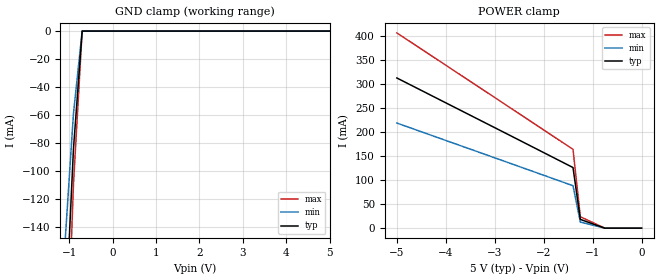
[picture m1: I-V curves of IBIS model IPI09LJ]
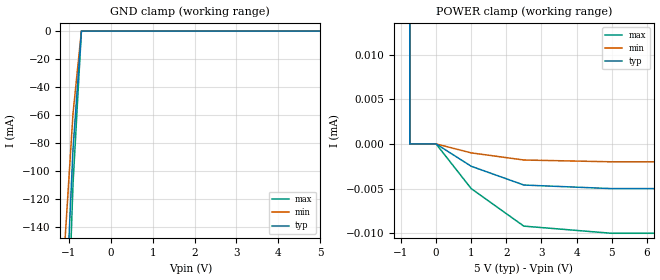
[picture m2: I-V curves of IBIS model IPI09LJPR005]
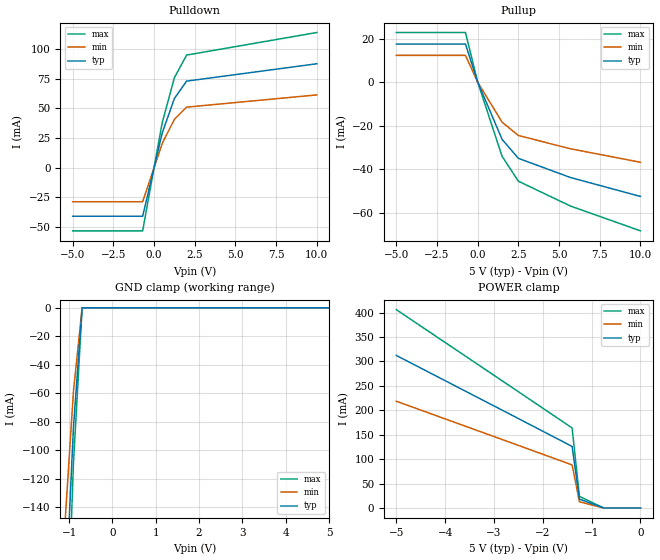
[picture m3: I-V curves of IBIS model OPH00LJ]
[IBIS Ver]   2.1
[File name]   act8997.ibs
[File Rev]   1.0   | from silicon model only
[Date]   97318
[Source]   Silicon-level model at Texas Instruments (ALEY)
[Notes]
   SCAN PATH LINKERS WITH 4-BIT IDENTIFICATION BUSES
   SCAN-CONTROLLED IEEE STD 1149.1 (JTAG) TAP CONCATENATORS
   Release 1.0) 97318 ALEY - initial release
   includes DCO open-drain (_OD) and DCO 3-state (_TS)
   includes all available commercial packages:
   DW=28SOIC (no-coupling model)
   NT=28PDIP (no-coupling model)
[Disclaimer]
   Property of Texas Instruments Incorporated.  Unauthorized
   reproduction and/or distribution is strictly prohibited.
   This product is protected under copyright law.
   Created 1997, (C) Copyright 1997, Texas Instruments Incorporated.
   All Rights Reserved
   UNLESS THERE IS A SIGNED, WRITTEN AGREEMENT TO THE
   CONTRARY, TEXAS INSTRUMENTS ("TI") IS PROVIDING THE IBIS
   MODELS "AS IS" AND WITHOUT ANY WARRANTY, EXPRESSED OR
   IMPLIED.  TI assumes no liability for:
   1) the accuracy of the IBIS models provided to your
   company;
   2) the proper functioning of these IBIS models in your
   design or for any resulting applications; or
   3) infringement of patents, copyrights or intellectual
   property rights resulting from your use of these IBIS
   models.
   TI provides IBIS Models as a service to our customers.
   You and your company shall not distribute, sell or give
   these models to anyone else without prior written
   permission from TI.
   TI reserves the right to make changes to our products or
   to discontinue any semiconductor product or service
   without notice, and advises our customers to obtain the
   latest version of relevant information to verify, before
   placing orders, that the information being relied on is
   current.
   Please be aware that your receipt and use of the IBIS
   information provided shall serve as acceptance of these
   terms and conditions.  If you do not accept these terms,
   you should return or destroy the IBIS models and any
   other accompanying information immediately.
[Component]   SN74ACT8997DW_OD
[Manufacturer]  Texas Instruments
[Package]
| 28-pin SOIC (suffix = DW)
| variable   typ   min   max
R_pkg   100m   NA   NA
L_pkg   7n   NA   NA
C_pkg   1p   NA   NA
[Pin]   signal_name   model_name   R_pin   L_pin   C_pin
1   DCO   OPHA1LJ   NA   8.15N   1.06P
2   MCO   OPH00LJ   NA   6.75N   0.98P
3   DTDO1   OPH03LJ   NA   5.49N   0.92P
4   DTDO2   OPH03LJ   NA   4.44N   0.64P
5   DTDO3   OPH03LJ   NA   3.74N   0.55P
6   DTDO4   OPH03LJ   NA   3.14N   0.46P
7   GND   GND   NA   2.85N   0.40P
8   DTMS1   OPHB3LJ   NA   2.85N   0.40P
9   DTMS2   OPHB3LJ   NA   3.14N   0.46P
10   DTMS3   OPHB3LJ   NA   3.74N   0.55P
11   DTMS4   OPHB3LJ   NA   4.44N   0.64P
12   DTCK   OPJE3LJ   NA   5.49N   0.92P
13   TDO   OPH03LJ   NA   6.75N   0.98P
14   TMS   IPI09LJPR005   NA   8.15N   1.06P
15   TCK   IPI09LJ   NA   8.15N   1.06P
16   TDI   IPI09LJPR005   NA   6.75N   0.98P
17   DTDI4   IPI09LJPR005   NA   5.49N   0.92P
18   DTDI3   IPI09LJPR005   NA   4.44N   0.64P
19   DTDI2   IPI09LJPR005   NA   3.74N   0.55P
20   DTDI1   IPI09LJPR005   NA   3.14N   0.46P
21   VCC   POWER   NA   2.85N   0.40P
22   ID4   IPI09LJ   NA   2.85N   0.40P
23   ID3   IPI09LJ   NA   3.14N   0.46P
24   ID2   IPI09LJ   NA   3.74N   0.55P
25   ID1   IPI09LJ   NA   4.44N   0.64P
26   TRSTN   IPI09LJPR005   NA   5.49N   0.92P
27   MCI   IPI09LJ   NA   6.75N   0.98P
28   DCI   IPI09LJ   NA   8.15N   1.06P
[Component]   SN74ACT8997DW_TS
[Manufacturer]  Texas Instruments
[Package]
| 28-pin SOIC (suffix = DW)
| variable   typ   min   max
R_pkg   100m   NA   NA
L_pkg   7n   NA   NA
C_pkg   1p   NA   NA
[Pin]   signal_name   model_name   R_pin   L_pin   C_pin
1   DCO   OPHA3LJ   NA   8.15N   1.06P
2   MCO   OPH00LJ   NA   6.75N   0.98P
3   DTDO1   OPH03LJ   NA   5.49N   0.92P
4   DTDO2   OPH03LJ   NA   4.44N   0.64P
5   DTDO3   OPH03LJ   NA   3.74N   0.55P
6   DTDO4   OPH03LJ   NA   3.14N   0.46P
7   GND   GND   NA   2.85N   0.40P
8   DTMS1   OPHB3LJ   NA   2.85N   0.40P
9   DTMS2   OPHB3LJ   NA   3.14N   0.46P
10   DTMS3   OPHB3LJ   NA   3.74N   0.55P
11   DTMS4   OPHB3LJ   NA   4.44N   0.64P
12   DTCK   OPJE3LJ   NA   5.49N   0.92P
13   TDO   OPH03LJ   NA   6.75N   0.98P
14   TMS   IPI09LJPR005   NA   8.15N   1.06P
15   TCK   IPI09LJ   NA   8.15N   1.06P
16   TDI   IPI09LJPR005   NA   6.75N   0.98P
17   DTDI4   IPI09LJPR005   NA   5.49N   0.92P
18   DTDI3   IPI09LJPR005   NA   4.44N   0.64P
19   DTDI2   IPI09LJPR005   NA   3.74N   0.55P
20   DTDI1   IPI09LJPR005   NA   3.14N   0.46P
21   VCC   POWER   NA   2.85N   0.40P
22   ID4   IPI09LJ   NA   2.85N   0.40P
23   ID3   IPI09LJ   NA   3.14N   0.46P
24   ID2   IPI09LJ   NA   3.74N   0.55P
25   ID1   IPI09LJ   NA   4.44N   0.64P
26   TRSTN   IPI09LJPR005   NA   5.49N   0.92P
27   MCI   IPI09LJ   NA   6.75N   0.98P
28   DCI   IPI09LJ   NA   8.15N   1.06P
[Component]   SN74ACT8997NT_OD
[Manufacturer]  Texas Instruments
[Package]
| 28-pin PDIP (suffix = NT)
| variable   typ   min   max
R_pkg   100m   NA   NA
L_pkg   10n   NA   NA
C_pkg   2p   NA   NA
[Pin]   signal_name   model_name   R_pin   L_pin   C_pin
1   DCO   OPHA1LJ   NA   15.08N   2.15P
2   MCO   OPH00LJ   NA   12.33N   1.86P
3   DTDO1   OPH03LJ   NA   9.57N   1.70P
4   DTDO2   OPH03LJ   NA   6.90N   1.29P
5   DTDO3   OPH03LJ   NA   5.45N   0.95P
6   DTDO4   OPH03LJ   NA   3.89N   0.61P
7   GND   GND   NA   2.75N   0.43P
8   DTMS1   OPHB3LJ   NA   2.75N   0.43P
9   DTMS2   OPHB3LJ   NA   3.89N   0.61P
10   DTMS3   OPHB3LJ   NA   5.45N   0.95P
11   DTMS4   OPHB3LJ   NA   6.90N   1.29P
12   DTCK   OPJE3LJ   NA   9.57N   1.70P
13   TDO   OPH03LJ   NA   12.33N   1.86P
14   TMS   IPI09LJPR005   NA   15.08N   2.15P
15   TCK   IPI09LJ   NA   15.08N   2.15P
16   TDI   IPI09LJPR005   NA   12.33N   1.86P
17   DTDI4   IPI09LJPR005   NA   9.57N   1.70P
18   DTDI3   IPI09LJPR005   NA   6.90N   1.29P
19   DTDI2   IPI09LJPR005   NA   5.45N   0.95P
20   DTDI1   IPI09LJPR005   NA   3.89N   0.61P
21   VCC   POWER   NA   2.75N   0.43P
22   ID4   IPI09LJ   NA   2.75N   0.43P
23   ID3   IPI09LJ   NA   3.89N   0.61P
24   ID2   IPI09LJ   NA   5.45N   0.95P
25   ID1   IPI09LJ   NA   6.90N   1.29P
26   TRSTN   IPI09LJPR005   NA   9.57N   1.70P
27   MCI   IPI09LJ   NA   12.33N   1.86P
28   DCI   IPI09LJ   NA   15.08N   2.15P
[Component]   SN74ACT8997NT_TS
[Manufacturer]  Texas Instruments
[Package]
| 28-pin PDIP (suffix = NT)
| variable   typ   min   max
R_pkg   100m   NA   NA
L_pkg   10n   NA   NA
C_pkg   2p   NA   NA
[Pin]   signal_name   model_name   R_pin   L_pin   C_pin
1   DCO   OPHA3LJ   NA   15.08N   2.15P
2   MCO   OPH00LJ   NA   12.33N   1.86P
3   DTDO1   OPH03LJ   NA   9.57N   1.70P
4   DTDO2   OPH03LJ   NA   6.90N   1.29P
5   DTDO3   OPH03LJ   NA   5.45N   0.95P
6   DTDO4   OPH03LJ   NA   3.89N   0.61P
7   GND   GND   NA   2.75N   0.43P
8   DTMS1   OPHB3LJ   NA   2.75N   0.43P
9   DTMS2   OPHB3LJ   NA   3.89N   0.61P
10   DTMS3   OPHB3LJ   NA   5.45N   0.95P
11   DTMS4   OPHB3LJ   NA   6.90N   1.29P
12   DTCK   OPJE3LJ   NA   9.57N   1.70P
13   TDO   OPH03LJ   NA   12.33N   1.86P
14   TMS   IPI09LJPR005   NA   15.08N   2.15P
15   TCK   IPI09LJ   NA   15.08N   2.15P
16   TDI   IPI09LJPR005   NA   12.33N   1.86P
17   DTDI4   IPI09LJPR005   NA   9.57N   1.70P
18   DTDI3   IPI09LJPR005   NA   6.90N   1.29P
19   DTDI2   IPI09LJPR005   NA   5.45N   0.95P
20   DTDI1   IPI09LJPR005   NA   3.89N   0.61P
21   VCC   POWER   NA   2.75N   0.43P
22   ID4   IPI09LJ   NA   2.75N   0.43P
23   ID3   IPI09LJ   NA   3.89N   0.61P
24   ID2   IPI09LJ   NA   5.45N   0.95P
25   ID1   IPI09LJ   NA   6.90N   1.29P
26   TRSTN   IPI09LJPR005   NA   9.57N   1.70P
27   MCI   IPI09LJ   NA   12.33N   1.86P
28   DCI   IPI09LJ   NA   15.08N   2.15P
| Models and submodels in the file (8): IPI09LJ (Input), IPI09LJPR005 (Input), OPH00LJ (Output), OPH03LJ (3-state), OPHA1LJ (Open_drain), OPHA3LJ (3-state), OPHB3LJ (3-state), OPJE3LJ (3-state)
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[Model]   IPI09LJ
| TTL-compatible input buffer with hysteresis
| IP (97318 ALEY)
| BP (97318 ALEY)
Model_type   Input
Polarity   Non-Inverting
| Signals   DCI, ID1-4, MCI, TCK
Vinl = 0.8V
Vinh = 2.0V
| variable   typ   min   max
C_comp   6pF   NA   NA
| variable   typ   min   max
[Voltage range]   5.0V   4.5V   5.5V
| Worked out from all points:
|   GND clamp passes 1 mA (typ) near -0.70 V on its own axis
[power_clamp]
|   50C:5V:   100C:4.5V:weak  0C:5.5V:strong
| Voltage   I(typ)   I(min)   I(max)
-5V       312.2mA    218.5mA    405.9mA
-2.75V    196mA      137.2mA    254.8mA
-1.4V     126mA      88.2mA     163.8mA
-1.25V    18.2mA     12.7mA     23.7mA
-750mV    0A         0A         0A
0V        0A         0A         0A
[gnd_clamp]
|   50C:5V:   100C:4.5V:weak  0C:5.5V:strong
| Voltage   I(typ)   I(min)   I(max)
-5V       -2.8A      -2A        -3.6A
-900mV    -84mA      -58.8mA    -109.2mA
-700mV    0A         0A         0A
0V        0A         0A         0A
5V        0A         0A         0A
[Model]   IPI09LJPR005
| TTL-compatible input buffer with hysteresis
|   and 5-uA pull-up active terminator
| IP (97318 ALEY)
| BP (97318 ALEY)
| PR (97318 ALEY)
Model_type   Input
Polarity   Non-Inverting
| Signals   DCI, ID1-4, MCI, TCK
Vinl = 0.8V
Vinh = 2.0V
| variable   typ   min   max
C_comp   6pF   NA   NA
| variable   typ   min   max
[Voltage range]   5.0V   4.5V   5.5V
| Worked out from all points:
|   GND clamp passes 1 mA (typ) near -0.70 V on its own axis
[power_clamp]
|   50C:5V:   100C:4.5V:weak  0C:5.5V:strong
| Voltage   I(typ)   I(min)   I(max)
-5V       312.2mA    218.5mA    405.9mA
-2.75V    196mA      137.2mA    254.8mA
-1.4V     126mA      88.2mA     163.8mA
-1.25V    18.2mA     12.7mA     23.7mA
-750mV    0A         0A         0A
0V        0A         0A         0A
1V        -2.5uA     -1uA       -5uA
2.5V      -4.6uA     -1.8uA     -9.2uA
5V        -5uA       -2uA       -10uA
10V       -5uA       -2uA       -10uA
[gnd_clamp]
|   50C:5V:   100C:4.5V:weak  0C:5.5V:strong
| Voltage   I(typ)   I(min)   I(max)
-5V       -2.8A      -2A        -3.6A
-900mV    -84mA      -58.8mA    -109.2mA
-700mV    0A         0A         0A
0V        0A         0A         0A
5V        0A         0A         0A
[Model]   OPH00LJ
| 10-mA totem-pole CMOS/TTL output buffer with 0.125 di/dt
| OP (97318 ALEY)
| BP (97318 ALEY)
Model_type   Output
Polarity   Non-Inverting
| Signals   MCO
| variable   typ   min   max
C_comp   10pF   NA   NA
| variable   typ   min   max
[Voltage range]   5.0V   4.5V   5.5V
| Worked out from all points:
|   slope of the pulldown table from 0 to 0.75 V, typ, clamps not added: 19.3 ohm
|   slope of the pullup table from 0 to 0.75 V, typ, clamps not added: 57 ohm
|   GND clamp passes 1 mA (typ) near -0.70 V on its own axis
[pullup]
|   50C:5V:   100C:4.5V:weak  0C:5.5V:strong
| Voltage   I(typ)   I(min)   I(max)
-5V       17.5mA     12.3mA     22.8mA
-2.75V    17.5mA     12.3mA     22.8mA
-1.4V     17.5mA     12.3mA     22.8mA
-1.25V    17.5mA     12.3mA     22.8mA
-750mV    17.5mA     12.3mA     22.8mA
0V        0A         0A         0A
1.5V      -26.3mA    -18.4mA    -34.1mA
2.5V      -35mA      -24.5mA    -45.5mA
5.7V      -43.8mA    -30.6mA    -56.9mA
10V       -52.5mA    -36.8mA    -68.3mA
[pulldown]
|   50C:5V:   100C:4.5V:weak  0C:5.5V:strong
| Voltage   I(typ)   I(min)   I(max)
-5V       -40.8mA    -28.6mA    -53.1mA
-900mV    -40.8mA    -28.6mA    -53.1mA
-700mV    -40.8mA    -28.6mA    -53.1mA
-500mV    -29.2mA    -20.4mA    -37.9mA
0V        0A         0A         0A
500mV     29.2mA     20.4mA     37.9mA
1.25V     58.3mA     40.8mA     75.8mA
2V        72.9mA     51mA       94.8mA
10V       87.5mA     61.3mA     113.8mA
[power_clamp]
|   50C:5V:   100C:4.5V:weak  0C:5.5V:strong
| Voltage   I(typ)   I(min)   I(max)
-5V       312.2mA    218.5mA    405.9mA
-2.75V    196mA      137.2mA    254.8mA
-1.4V     126mA      88.2mA     163.8mA
-1.25V    18.2mA     12.7mA     23.7mA
-750mV    0A         0A         0A
0V        0A         0A         0A
[gnd_clamp]
|   50C:5V:   100C:4.5V:weak  0C:5.5V:strong
| Voltage   I(typ)   I(min)   I(max)
-5V       -2.8A      -2A        -3.6A
-900mV    -84mA      -58.8mA    -109.2mA
-700mV    0A         0A         0A
0V        0A         0A         0A
5V        0A         0A         0A
[ramp]
| variable   typ   min   max
dV/dt_r   1.2/2.25e-9   0.9/3.375e-9   1.5/1.5e-9
dV/dt_f   1.8/2e-9   1.5/3e-9   2.1/1.33e-9
